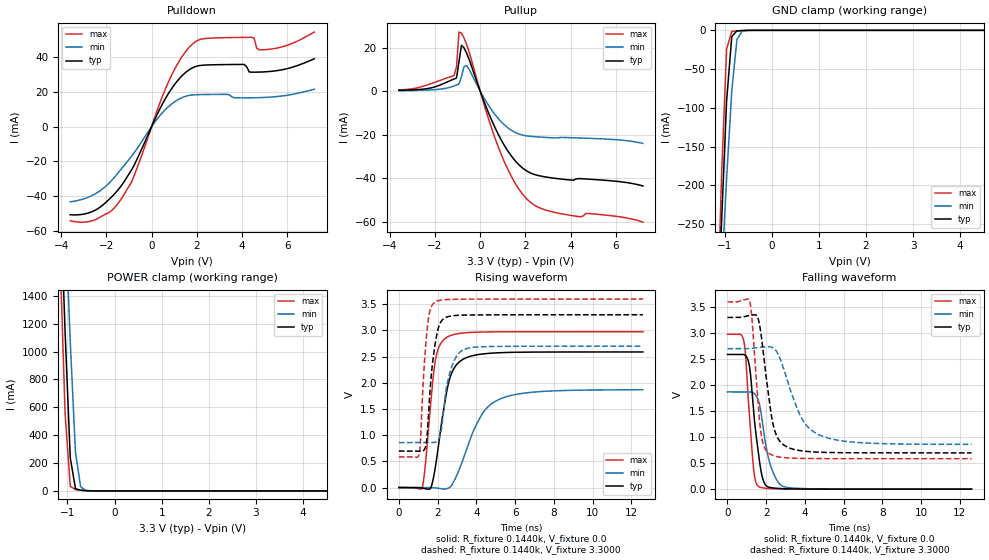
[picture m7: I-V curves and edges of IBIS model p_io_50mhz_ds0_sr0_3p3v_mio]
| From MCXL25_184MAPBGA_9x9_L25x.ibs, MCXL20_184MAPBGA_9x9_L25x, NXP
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[Model] p_io_50mhz_ds0_sr0_3p3v_mio
|   Model p_io_50mhz_ds0_sr0_3p3v_mio
| This model was characterised for following simulation conditions:
| External (pad) voltage:
|   - Typ: 3.3V,   - Min: 2.7V,   - Max: 3.6V
| Library cells for typ/min/max conditions are connected as defined below:
|  pad - External Pad
|  ipp_do_lv - Core Input
|  ipp_obe_lv - Output Buffer Enable
|  IOGC - NC
|  REFH3V3 - REFH3V3
|  REFL3V3 - REFL3V3
|  ZI - NC
|  abut_ncal_vddio[1] - vddio
|  abut_ncal_vddio[2] - vddio
|  abut_ncal_vddio[3] - vssio
|  abut_ncal_vddio[4] - vddio
|  abut_ncal_vddio[5] - vddio
|  abut_ncal_vddio[6] - vssio
|  abut_pcal_vddio[1] - vssio
|  abut_pcal_vddio[2] - vssio
|  abut_pcal_vddio[3] - vddio
|  abut_pcal_vddio[4] - vssio
|  abut_pcal_vddio[5] - vssio
|  abut_pcal_vddio[6] - vddio
|  ipp_do_1p8v - ipp_do_1p8v
|  ipp_dse_lv - 0
|  ipp_eftd_lv - NC
|  ipp_ina_mux_vddio - NC
|  ipp_ina_mux_vddio[0] - NC
|  ipp_ina_mux_vddio[1] - NC
|  ipp_ina_r0_vddio - NC
|  ipp_ina_r0a_vddio - NC
|  ipp_ina_r0b_vddio - NC
|  ipp_ina_r0c_vddio - NC
|  ipp_ina_r0d_vddio - NC
|  ipp_ina_r0e_vddio - NC
|  ipp_ina_r0f_vddio - NC
|  ipp_ina_r300_vddio - NC
|  ipp_ina_r300a_vddio - NC
|  ipp_ina_r300b_vddio - NC
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Model_type I/O
Polarity   Non-Inverting
Enable   Active-High
Vinl =   0.9900V
Vinh =   2.3100V
Vmeas =  1.6500V
Cref =   30.0000pF
Rref =   1.0000M
Vref =   3.3000V
C_comp   1.4363pF   1.3758pF   1.5227pF
|C_comp_pullup   0.7191pF   0.7514pF   0.6972pF
|C_comp_pulldown   0.6284pF   0.6829pF   0.5891pF
[Model Spec]
| variable   typ   min   max
Vinh   2.3100V   1.8900V   2.5200V
Vinl   0.9900V   0.8100V   1.0800V
[Temperature Range]   25.0000   0.1250k   -40.0000
[Voltage Range]   3.3000V   2.7000V   3.6000V
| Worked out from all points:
|   slope of the pulldown table from 0 to 0.495 V, typ, clamps not added: 36.8 ohm
|   slope of the pullup table from 0 to 0.495 V, typ, clamps not added: 37.8 ohm
|   GND clamp passes 1 mA (typ) near -0.74 V on its own axis
|   POWER clamp passes 1 mA (typ) near -0.54 V on its own axis
|   rising waveform, R_fixture 0.1440k, V_fixture 0.0: 20-80 % time 680ps typ, 1.33ns min, 455ps max; typ from 0 V to 2.59 V
|   rising waveform, R_fixture 0.1440k, V_fixture 3.3000: 20-80 % time 390ps typ, 520ps min, 299ps max; typ from 0.697 V to 3.3 V
|   falling waveform, R_fixture 0.1440k, V_fixture 0.0: 20-80 % time 436ps typ, 577ps min, 326ps max; typ from 2.59 V to 0 V
|   falling waveform, R_fixture 0.1440k, V_fixture 3.3000: 20-80 % time 570ps typ, 1.19ns min, 369ps max; typ from 3.3 V to 0.697 V
[Pulldown]
|Voltage   I(typ)   I(min)   I(max)
-3.6V     -50.71mA   -43.27mA   -54.18mA
-2.5V     -48.1mA    -38.69mA   -53.56mA
-1.4V     -35.02mA   -25.26mA   -42.7mA
-850mV    -24.18mA   -16.32mA   -30.69mA
800mV     20.23mA    12.14mA    27.32mA
1.9V      34.45mA    18.38mA    48.57mA
4.1V      35.83mA    16.63mA    51.44mA
4.43V     31.42mA    16.66mA    51.52mA
4.54V     31.41mA    16.69mA    50.94mA
4.65V     31.42mA    16.71mA    45.28mA
5.09V     31.67mA    16.92mA    44.44mA
7.2V      39.12mA    21.58mA    54.49mA
[Pullup]
|Voltage   I(typ)   I(min)   I(max)
-3.6V     390.2uA    234.7uA    600.5uA
-1.16V    5.607mA    2.418mA    7.152mA
-1.05V    6.059mA    2.87mA     11.01mA
-940mV    13.57mA    3.339mA    27.22mA
-830mV    21.13mA    6.682mA    26.77mA
-720mV    20.02mA    11.25mA    24.57mA
-610mV    17.72mA    11.8mA     21.82mA
820mV     -20.27mA   -12.85mA   -26.19mA
1.48V     -31.2mA    -18.62mA   -41.17mA
2.03V     -36.53mA   -20.52mA   -49.25mA
3.46V     -40.29mA   -21.45mA   -56.15mA
7.2V      -43.65mA   -24.03mA   -60.31mA
[GND_clamp]
|Voltage   I(typ)   I(min)   I(max)
-3.6V     -4.967A    -3.834A    -6.451A
-1.18V    -432.4mA   -454.2mA   -428.7mA
-1.07V    -252.8mA   -319.9mA   -193.4mA
-960mV    -91.54mA   -192mA     -24.27mA
-850mV    -8.013mA   -77.89mA   -1.462mA
-740mV    -731.9uA   -11.92mA   -724.8uA
-630mV    -284.5uA   -928.5uA   -315.1uA
-300mV    -508.9nA   -3.038uA   -108.6nA
7.2V      0A         0A         0A
[POWER_clamp]
|Voltage   I(typ)   I(min)   I(max)
-3.6V     26.34A     23.98A     28.82A
-1.16V    2.208A     2.937A     1.722A
-1.05V    1.14A      1.999A     556.4mA
-940mV    237.9mA    1.069A     33.46mA
-830mV    16.33mA    277.1mA    9.216mA
-720mV    4.663mA    29.2mA     4.86mA
-610mV    1.877mA    3.923mA    1.821mA
7.2V      0A         0A         0A
[Ramp]
| variable   typ   min   max
dV/dt_r  1.5537/0.6797n   1.1207/1.3303n   1.7857/0.4551n
dV/dt_f  1.5618/0.5697n   1.1038/1.1884n   1.8085/0.3687n
R_load = 0.1440k
[Rising Waveform]
R_fixture= 0.1440k
V_fixture= 0.0
V_fixture_min= 0.0
V_fixture_max= 0.0
|time   V(typ)   V(min)   V(max)
0s        4.584nV    239.2nV    15.27nV
1.207ns   -10.31mV   -152.2uV   -5.06mV
1.359ns   -20.54mV   283uV      401mV
1.632ns   -17.89mV   593.1uV    1.571V
1.856ns   326.7mV    -6.286mV   2.363V
2.45ns    1.792V     -25.14mV   2.863V
3.122ns   2.401V     347.8mV    2.943V
4.196ns   2.546V     1.34V      2.97V
5.084ns   2.573V     1.668V     2.974V
12.6ns    2.589V     1.868V     2.976V
[Rising Waveform]
R_fixture= 0.1440k
V_fixture= 3.3000
V_fixture_min= 2.7000
V_fixture_max= 3.6000
|time   V(typ)   V(min)   V(max)
0s        696.8mV    859.1mV    585.8mV
1.051ns   696.9mV    859mV      643.9mV
1.344ns   743.4mV    859.5mV    2.516V
1.469ns   1.041V     860.6mV    3.055V
1.66ns    2.086V     859.6mV    3.442V
1.862ns   2.716V     862.5mV    3.539V
2.152ns   3.155V     1.022V     3.579V
2.666ns   3.275V     2.236V     3.594V
3.357ns   3.294V     2.636V     3.598V
12.6ns    3.3V       2.7V       3.6V
[Falling Waveform]
R_fixture= 0.1440k
V_fixture= 0.0
V_fixture_min= 0.0
V_fixture_max= 0.0
|time   V(typ)   V(min)   V(max)
0s        2.589V     1.869V     2.976V
849.6ps   2.588V     1.869V     2.836V
938.1ps   2.566V     1.868V     2.556V
1.139ns   2.354V     1.87V      1.408V
1.336ns   1.535V     1.851V     429.8mV
1.61ns    650.5mV    1.686V     49.59mV
1.863ns   153.6mV    1.118V     22.24mV
2.186ns   32.66mV    497.6mV    11.49mV
2.889ns   9.439mV    51.56mV    3.285mV
12.6ns    39.08uV    81.11uV    27.19uV
[Falling Waveform]
R_fixture= 0.1440k
V_fixture= 3.3000
V_fixture_min= 2.7000
V_fixture_max= 3.6000
|time   V(typ)   V(min)   V(max)
0s        3.3V       2.7V       3.6V
1.149ns   3.336V     2.701V     3.611V
1.525ns   3.327V     2.721V     1.923V
1.718ns   3.017V     2.728V     1.108V
2.193ns   1.596V     2.737V     676.2mV
2.462ns   1.098V     2.683V     634.3mV
2.798ns   882.7mV    2.427V     610.3mV
3.784ns   738.3mV    1.395V     590.7mV
4.717ns   710.3mV    1.047V     587.4mV
12.6ns    697mV      860.3mV    585.9mV
